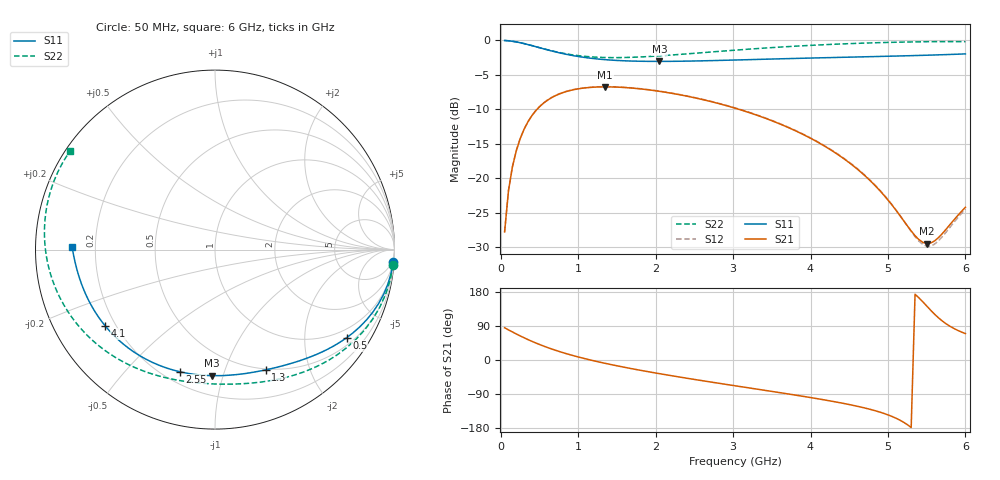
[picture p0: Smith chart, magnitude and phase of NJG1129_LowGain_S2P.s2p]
!S parameter
! Frequency  S11  S21  S12  S22
# HZ  S  DB R 50
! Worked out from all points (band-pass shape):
!   120 points, 50 MHz to 6 GHz, reference 50 ohm
!   highest |S21| = -6.75 dB at 1.35 GHz (marker M1); lowest = -29.4 dB at 5.5 GHz (marker M2)
!   |S21| within 3 dB of the highest: 490.2 MHz to 3.001 GHz (2.511 GHz wide, 144 % of centre)
!   lowest |S11| = -3.1 dB at 2.05 GHz (marker M3), VSWR 5.72, Z = 16.6 - j45.9 ohm
!   |S11| at or under -10 dB: nowhere
!   |S22| runs from -2.5 to 0.0 dB; largest |S21 - S12| = 0.0022
!   S11 on the Smith chart (normalised r, x): 50 MHz: 2, -30; 500 MHz: 0.71, -3.14; 1.3 GHz: 0.49, -1.39; 2.55 GHz: 0.26, -0.72; 4.1 GHz: 0.16, -0.31; 6 GHz: 0.11, +0.01
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5e7  -0.04 -3.8  -27.75 85.0  -27.73 85.0  -0.04 -5.0
1e8  -0.09 -7.6  -21.80 79.5  -21.77 79.5  -0.08 -9.8
1.5e8  -0.15 -11.3  -18.38 74.1  -18.35 74.1  -0.15 -14.7
2e8  -0.25 -14.9  -16.03 68.8  -16.01 68.8  -0.24 -19.4
3.5e8  -0.63 -25.0  -11.84 54.1  -11.82 54.1  -0.62 -32.6
5e8  -1.08 -33.8  -9.64 41.0  -9.61 41.0  -1.07 -44.3
7.5e8  -1.81 -46.1  -7.81 22.8  -7.78 22.9  -1.76 -60.5
1.05e9  -2.44 -58.2  -6.96 5.4  -6.93 5.5  -2.30 -76.0
1.3e9  -2.77 -67.2  -6.76 -6.6  -6.73 -6.5  -2.49 -87.0
1.35e9  -2.82 -68.9  -6.75 -8.9  -6.73 -8.8  -2.51 -89.0
2.05e9  -3.07 -91.4  -7.40 -36.1  -7.37 -35.9  -2.27 -114.0
2.55e9  -3.00 -106.2  -8.45 -52.9  -8.41 -52.7  -1.85 -129.3
3.05e9  -2.86 -119.9  -9.92 -68.8  -9.88 -68.5  -1.42 -143.4
3.55e9  -2.71 -132.5  -11.88 -84.5  -11.83 -84.1  -1.04 -156.5
4.05e9  -2.57 -144.2  -14.49 -100.8  -14.44 -100.2  -0.72 -169.0
4.1e9  -2.56 -145.3  -14.80 -102.5  -14.74 -101.9  -0.69 -170.2
4.65e9  -2.42 -156.9  -19.09 -124.2  -19.02 -123.2  -0.44 176.8
5.05e9  -2.31 -164.6  -23.83 -148.8  -23.77 -146.9  -0.31 167.5
5.35e9  -2.22 -170.0  -28.30 173.5  -28.44 176.5  -0.24 160.6
5.5e9  -2.17 -172.6  -29.44 142.6  -29.82 145.2  -0.22 157.2
5.65e9  -2.12 -175.2  -28.60 111.7  -29.07 112.7  -0.21 153.7
6e9  -1.98 179.1  -24.19 69.7  -24.46 69.2  -0.21 145.6
